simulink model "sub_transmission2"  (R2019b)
settings: Solver=ode23t  StartTime=0.0  StopTime=10.0  RelTol=1e-3
libraries: simulink x3

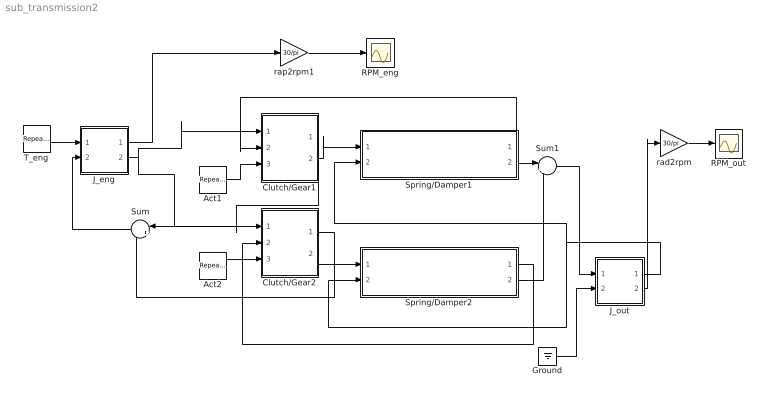
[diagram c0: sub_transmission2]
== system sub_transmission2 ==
  Act1 : simulink/Sources/Repeating Sequence  rep_seq_t=[0 0.2 5 5.2 10]  rep_seq_y=[0 1 1 0 0]
  Act2 : simulink/Sources/Repeating Sequence  rep_seq_t=[0 5 5.2 10]  rep_seq_y=[0 0 1 1]
  Clutch/Gear1 : Subsystem
  Clutch/Gear2 : Subsystem
  Ground : Ground
  J_eng : Subsystem
  J_out : Subsystem
  RPM_eng : Scope
  RPM_out : Scope
  Spring/Damper1 : Subsystem
  Spring/Damper2 : Subsystem
  Sum : Sum  Inputs=|++
  Sum1 : Sum  Inputs=|++
  T_eng : simulink/Sources/Repeating Sequence  rep_seq_t=[0 2 10]  rep_seq_y=[0 250 250]
  rad2rpm : Gain  Gain=30/pi
  rap2rpm1 : Gain  Gain=30/pi
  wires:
  T_eng/1 -> J_eng/1(T1)
  Act1/1 -> Clutch/Gear1/3(APS)
  Act2/1 -> Clutch/Gear2/3(APS)
  Clutch/Gear1/1(T1) -> Sum/1
  Clutch/Gear2/1(T1) -> Sum/2
  Sum/1 -> J_eng/2(T2)
  Clutch/Gear1/2(w2) -> Spring/Damper1/1(w1)
  Clutch/Gear2/2(w2) -> Spring/Damper2/1(w1)
  Spring/Damper1/2(T2) -> Sum1/1
  Spring/Damper2/2(T2) -> Sum1/2
  Spring/Damper1/1(T1) -> Clutch/Gear1/2(T2)
  Spring/Damper2/1(T1) -> Clutch/Gear2/2(T2)
  Sum1/1 -> J_out/1(T1)
  J_out/1(w1) -> Spring/Damper2/2(w2), Spring/Damper1/2(w2)
  Ground/1 -> J_out/2(T2)
  J_eng/2(w2) -> Clutch/Gear1/1(w1), Clutch/Gear2/1(w1)
  rap2rpm1/1 -> RPM_eng/1
  J_out/2(w2) -> rad2rpm/1
  rad2rpm/1 -> RPM_out/1
  J_eng/1(w1) -> rap2rpm1/1

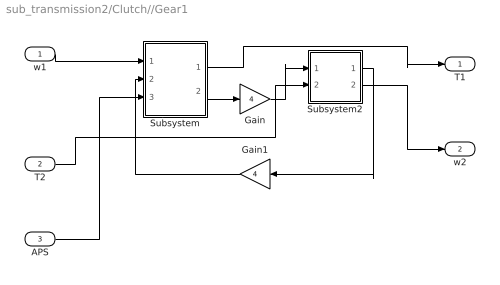
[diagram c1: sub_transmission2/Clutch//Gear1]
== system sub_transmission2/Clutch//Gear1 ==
  w1 : Inport
  T2 : Inport  Port=2
  APS : Inport  Port=3
  Gain : Gain  Gain=4
  Gain1 : Gain  Gain=4
  Subsystem : Subsystem
  Subsystem2 : Subsystem
  T1 : Outport
  w2 : Outport  Port=2
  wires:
  T2/1 -> Subsystem2/2(T2)
  Subsystem2/2(w2) -> w2/1
  Gain/1 -> Subsystem2/1(T1)
  Subsystem/1(T1) -> T1/1
  Gain1/1 -> Subsystem/2(w2)
  Subsystem2/1(w1) -> Gain1/1
  Subsystem/2(T2) -> Gain/1
  APS/1 -> Subsystem/3(APS)
  w1/1 -> Subsystem/1(w1)

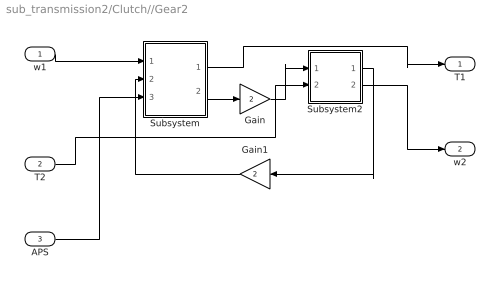
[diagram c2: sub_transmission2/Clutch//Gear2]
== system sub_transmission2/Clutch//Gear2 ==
  w1 : Inport
  T2 : Inport  Port=2
  APS : Inport  Port=3
  Gain : Gain  Gain=2
  Gain1 : Gain  Gain=2
  Subsystem : Subsystem
  Subsystem2 : Subsystem
  T1 : Outport
  w2 : Outport  Port=2
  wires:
  T2/1 -> Subsystem2/2(T2)
  Subsystem2/2(w2) -> w2/1
  Gain/1 -> Subsystem2/1(T1)
  Subsystem/1(T1) -> T1/1
  Gain1/1 -> Subsystem/2(w2)
  Subsystem2/1(w1) -> Gain1/1
  Subsystem/2(T2) -> Gain/1
  APS/1 -> Subsystem/3(APS)
  w1/1 -> Subsystem/1(w1)

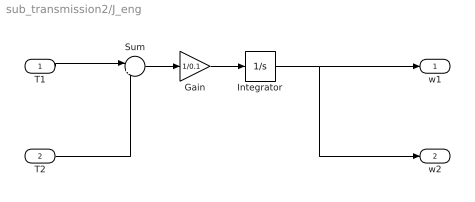
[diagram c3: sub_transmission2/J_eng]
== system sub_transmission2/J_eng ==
  T1 : Inport
  T2 : Inport  Port=2
  Gain : Gain  Gain=1/0.1
  Integrator : Integrator
  Sum : Sum  Inputs=|+-
  w1 : Outport
  w2 : Outport  Port=2
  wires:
  T1/1 -> Sum/1
  Integrator/1 -> w2/1, w1/1
  T2/1 -> Sum/2
  Sum/1 -> Gain/1
  Gain/1 -> Integrator/1

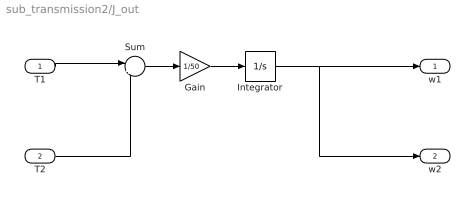
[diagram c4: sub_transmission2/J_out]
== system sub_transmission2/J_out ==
  T1 : Inport
  T2 : Inport  Port=2
  Gain : Gain  Gain=1/50
  Integrator : Integrator
  Sum : Sum  Inputs=|+-
  w1 : Outport
  w2 : Outport  Port=2
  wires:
  T1/1 -> Sum/1
  Integrator/1 -> w2/1, w1/1
  T2/1 -> Sum/2
  Sum/1 -> Gain/1
  Gain/1 -> Integrator/1

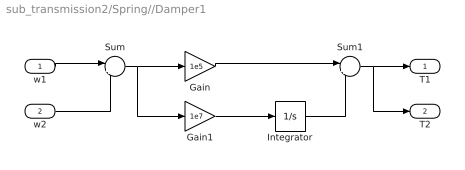
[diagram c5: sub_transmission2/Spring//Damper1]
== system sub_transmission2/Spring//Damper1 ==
  w1 : Inport
  w2 : Inport  Port=2
  Gain : Gain  Gain=1e5
  Gain1 : Gain  Gain=1e7
  Integrator : Integrator
  Sum : Sum  Inputs=|+-
  Sum1 : Sum  Inputs=|++
  T1 : Outport
  T2 : Outport  Port=2
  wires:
  w1/1 -> Sum/1
  w2/1 -> Sum/2
  Sum/1 -> Gain1/1, Gain/1
  Sum1/1 -> T2/1, T1/1
  Gain1/1 -> Integrator/1
  Gain/1 -> Sum1/1
  Integrator/1 -> Sum1/2

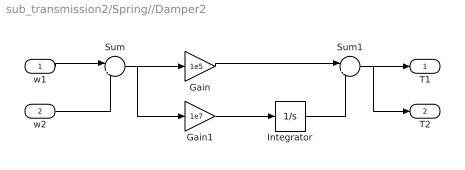
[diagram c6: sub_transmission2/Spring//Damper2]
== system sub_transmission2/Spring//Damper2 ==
  w1 : Inport
  w2 : Inport  Port=2
  Gain : Gain  Gain=1e5
  Gain1 : Gain  Gain=1e7
  Integrator : Integrator
  Sum : Sum  Inputs=|+-
  Sum1 : Sum  Inputs=|++
  T1 : Outport
  T2 : Outport  Port=2
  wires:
  w1/1 -> Sum/1
  w2/1 -> Sum/2
  Sum/1 -> Gain1/1, Gain/1
  Sum1/1 -> T2/1, T1/1
  Gain1/1 -> Integrator/1
  Gain/1 -> Sum1/1
  Integrator/1 -> Sum1/2

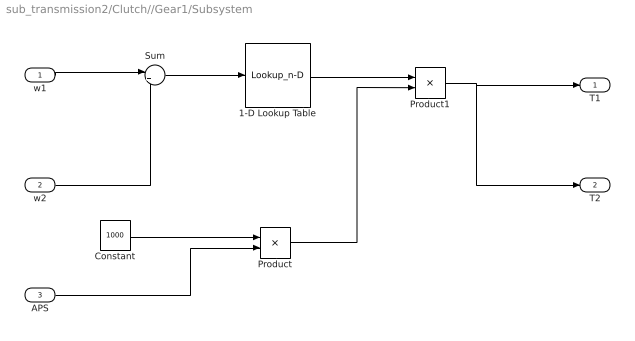
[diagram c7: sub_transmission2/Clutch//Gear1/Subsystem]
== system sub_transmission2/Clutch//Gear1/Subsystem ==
  w1 : Inport
  w2 : Inport  Port=2
  APS : Inport  Port=3
  1-D Lookup Table : Lookup_n-D  NumberOfTableDimensions=1  BreakpointsForDimension1=[-10:10]  Table=tanh(2*[-10:10])  InternalRulePriority=Speed  RndMeth=Simplest
  Constant : Constant  Value=1000
  Product : Product
  Product1 : Product
  Sum : Sum  Inputs=|+-
  T1 : Outport
  T2 : Outport  Port=2
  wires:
  Product1/1 -> T2/1, T1/1
  1-D Lookup Table/1 -> Product1/1
  APS/1 -> Product/2
  w2/1 -> Sum/2
  Product/1 -> Product1/2
  w1/1 -> Sum/1
  Sum/1 -> 1-D Lookup Table/1
  Constant/1 -> Product/1

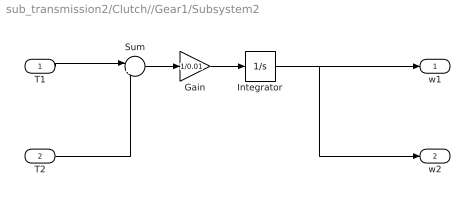
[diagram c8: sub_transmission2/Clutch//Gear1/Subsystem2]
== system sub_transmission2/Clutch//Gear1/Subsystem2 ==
  T1 : Inport
  T2 : Inport  Port=2
  Gain : Gain  Gain=1/0.01
  Integrator : Integrator
  Sum : Sum  Inputs=|+-
  w1 : Outport
  w2 : Outport  Port=2
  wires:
  T1/1 -> Sum/1
  Integrator/1 -> w2/1, w1/1
  T2/1 -> Sum/2
  Sum/1 -> Gain/1
  Gain/1 -> Integrator/1

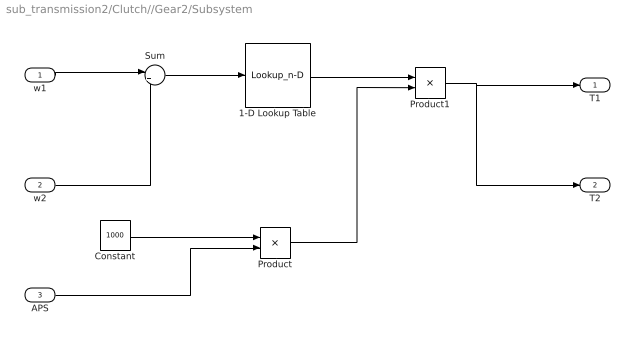
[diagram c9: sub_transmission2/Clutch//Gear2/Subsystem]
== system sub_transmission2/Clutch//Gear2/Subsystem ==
  w1 : Inport
  w2 : Inport  Port=2
  APS : Inport  Port=3
  1-D Lookup Table : Lookup_n-D  NumberOfTableDimensions=1  BreakpointsForDimension1=[-10:10]  Table=tanh(2*[-10:10])  InternalRulePriority=Speed  RndMeth=Simplest
  Constant : Constant  Value=1000
  Product : Product
  Product1 : Product
  Sum : Sum  Inputs=|+-
  T1 : Outport
  T2 : Outport  Port=2
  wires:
  Product1/1 -> T2/1, T1/1
  1-D Lookup Table/1 -> Product1/1
  APS/1 -> Product/2
  w2/1 -> Sum/2
  Product/1 -> Product1/2
  w1/1 -> Sum/1
  Sum/1 -> 1-D Lookup Table/1
  Constant/1 -> Product/1

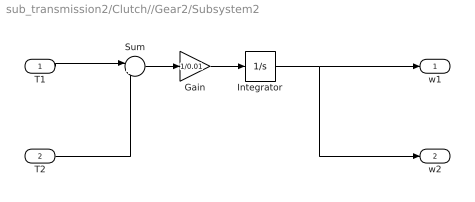
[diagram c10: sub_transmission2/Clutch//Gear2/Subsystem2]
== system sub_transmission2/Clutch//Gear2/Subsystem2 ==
  T1 : Inport
  T2 : Inport  Port=2
  Gain : Gain  Gain=1/0.01
  Integrator : Integrator
  Sum : Sum  Inputs=|+-
  w1 : Outport
  w2 : Outport  Port=2
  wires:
  T1/1 -> Sum/1
  Integrator/1 -> w2/1, w1/1
  T2/1 -> Sum/2
  Sum/1 -> Gain/1
  Gain/1 -> Integrator/1
